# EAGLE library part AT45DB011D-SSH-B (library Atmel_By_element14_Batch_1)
1-megabit Minimum DataFlash
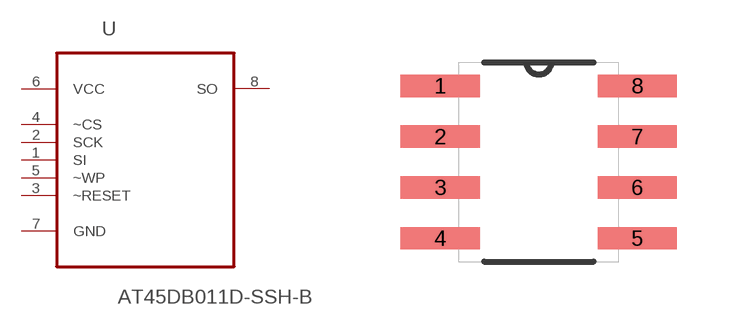
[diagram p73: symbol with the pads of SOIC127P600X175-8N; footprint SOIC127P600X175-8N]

Designator prefix U

## AT45DB011D-SSH-B (MPN: AT45DB011D-SSH-B; OC_FARNELL: 1715455; OC_NEWARK: 15R0319; PACKAGE: SOIC-8; SUPPLIER: Atmel)  [SOIC127P600X175-8N]
1  SI  in
2  SCK  in
3  ~RESET  in
4  ~CS  in
5  ~WP  in
6  VCC  pwr
7  GND  pas
8  SO  out

## Footprint SOIC127P600X175-8N (pad centres in mm)
smd 1.981 x 0.559: 1 -2.464,1.905; 2 -2.464,0.635; 3 -2.464,-0.635; 4 -2.464,-1.905; 5 2.464,-1.905; 6 2.464,-0.635; 7 2.464,0.635; 8 2.464,1.905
